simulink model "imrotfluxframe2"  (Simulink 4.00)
settings: Solver=ode45  StartTime=0.0  StopTime=1  MaxStep=2e-4  RelTol=1e-3  AbsTol=1e-3
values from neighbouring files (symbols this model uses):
  an = atan2(phiqr,phidr)    [imdefrotflux.m]
  Bm = 0.10    (= 0.1)    [IMabc2.m]    (also in imabcparam.m = 0.01; IMabcrun0.m = 0.01; IMabcrun1.m = 0.001; IMcur0.m = 1e-06)
  fr0 = [phidr phiqr]    [imdef0vec.m]    (also in imdef1vec.m; imdefrotflux.m = sqrt(phidr^2+phiqr^2); imdefSIvec1.m)
  fs0 = fs    [calc0.m]    (also in imdef0vec.m = [phids phiqs]; imdef1vec.m = [phids phiqs]; imdefrotflux.m = [fs0d fs0q]; imdefSIvec1.m = [phids phiqs])
  H = 0.60    (= 0.6)    [IMabc2.m]    (also in IMcur0.m = 0.3; imdef0vec.m = 0.3; imdef1vec.m = 0.3; imdef2vec.m = 0.3)
  Lm = eval(get(hLm,'String'))    [im3d.m]    (also in IMabc2.m = 4.5; imabcparam.m = 0.0847; IMabcrun0.m = 0.0847; IMabcrun1.m = 0.0847)
  Lrl = eval(get(hLr,'String'))    [im3d.m]    (also in IMabc2.m = 0.1; imabcparam.m = 0.0025; IMabcrun0.m = 0.0025; IMabcrun1.m = 0.0025)
  Lsl = eval(get(hLs,'String'))    [im3d.m]    (also in IMabc2.m = 0.1; imabcparam.m = 0.0025; IMabcrun0.m = 0.0025; IMabcrun1.m = 0.0025)
  n0 = 0.98    [imdef0vec.m]    (also in imdef1vec.m = 0.978; imdef2vec.m; imdefrotflux.m; imdefSIvec1.m = 0.95)
  Rr = input('Rotor resistance)[default = 2] =')    [Actac.m]    (also in im1phase.m = 0.3; im3d.m = eval(get(hRr,'String')); IMabc2.m = 0.02; imabcparam.m = 0.408)
  Rs = eval(get(hRs,'String'))    [im3d.m]    (also in IMabc2.m = 0.01; imabcparam.m = 0.531; IMabcrun0.m = 0.531; IMabcrun1.m = 0.531)
  Tl0 = Is*conj(Is)*Req    [imdef0vec.m]    (also in imdef1vec.m; imdef2vec.m = Lm*(I(2)*I(3)-I(1)*I(4)); imdefrotflux.m; imdefSIvec1.m = Te0/To)
  vs = 1.0    (= 1)    [imdef0vec.m]    (also in imdef1vec.m; imdef2vec.m; imdefrotflux.m; imdefSIvec1.m)
  wo = 2*pi*freq0    [calc0.m]    (also in IMabc2.m = 376.991118431; imabcparam.m = 376.991118431; IMabcrun0.m = 376.991118431; IMabcrun1.m = 376.991118431)
  ws = 1.0    (= 1)    [IMabc2.m]    (also in IMcur0.m; imdef0vec.m; imdef1vec.m; imdef2vec.m)

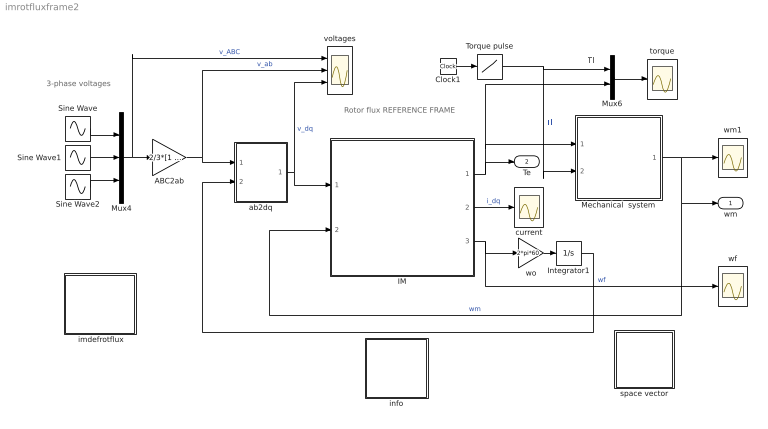
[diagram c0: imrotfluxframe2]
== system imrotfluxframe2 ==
  note: Rotor flux REFERENCE FRAME
  note: Tl
  note: 3-phase voltages
  " imdefrotflux" : Subsystem
  ABC2ab : Gain  Gain=2/3*[1 -0.5 -0.5;0 sqrt(3)/2 -sqrt(3)/2]  Multiplication=Matrix(K*u)  SaturateOnIntegerOverflow=on
  Clock1 : Clock
  IM : Subsystem
  Integrator1 : Integrator  ExternalReset=none  InitialConditionSource=internal  InitialCondition=0  LimitOutput=off  UpperSaturationLimit=inf  LowerSaturationLimit=-inf  ShowSaturationPort=off  ShowStatePort=off  AbsoluteTolerance=auto
  Mechanical  system : Subsystem
  Mux4 : Mux  Inputs=3
  Mux6 : Mux  Inputs=2
  Sine Wave : Sin  Amplitude=vs  Frequency=2*pi*ws*60  Phase=pi/2-an  SampleTime=0
  Sine Wave1 : Sin  Amplitude=vs  Frequency=2*pi*ws*60  Phase=pi/2-an-2*pi/3  SampleTime=0
  Sine Wave2 : Sin  Amplitude=vs  Frequency=2*pi*ws*60  Phase=pi/2-an+2*pi/3  SampleTime=0
  Torque pulse : Lookup  InputValues=[0 0.1 0.1 0.5 0.5 2]  OutputValues="[Tl0 Tl0  0 0 0.5 0.5]"
  ab2dq : Subsystem
  current : Scope
  info : Subsystem
  space vector : Subsystem
  torque : Scope
  voltages : Scope  NumInputPorts=3
  wf : Scope
  wm1 : Scope
  wo : Gain  Gain=2*pi*60  Multiplication=Element-wise(K.*u)  SaturateOnIntegerOverflow=on
  wm : Outport  Port=1
  Te : Outport  Port=2
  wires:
  Mux6/1 -> torque/1
  Torque pulse/1 -> Mux6/1, Mechanical  system/2(Tl)  "Tl"
  Mechanical  system/1(wm) -> wm1/1, IM/2(wm), wm/1  "wm"
  ab2dq/1(dq) -> IM/1(vs), voltages/3  "v_dq"
  Mux4/1 -> ABC2ab/1, voltages/1  "v_ABC"
  ABC2ab/1 -> ab2dq/1(ab), voltages/2  "v_ab"
  IM/2(is) -> current/1  "i_dq"
  IM/1(Te) -> Te/1, Mux6/2, Mechanical  system/1(Te)
  Sine Wave/1 -> Mux4/1
  Sine Wave1/1 -> Mux4/2
  Sine Wave2/1 -> Mux4/3
  Clock1/1 -> Torque pulse/1
  wo/1 -> Integrator1/1
  IM/3(wf) -> wo/1, wf/1  "wf"
  Integrator1/1 -> ab2dq/2(thetak)

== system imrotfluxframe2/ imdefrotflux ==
  note: Double click the block to enter the machine parameters and initial conditions and then run the simulation
  note: This demo simulates the running of an induction motor in steady-state when a sudden input change is effected: a)torque step changes at constant voltage excitation b) voltage input sag at constant frequency and load torque c)simultaneous step changes in voltage magnitude and frequency

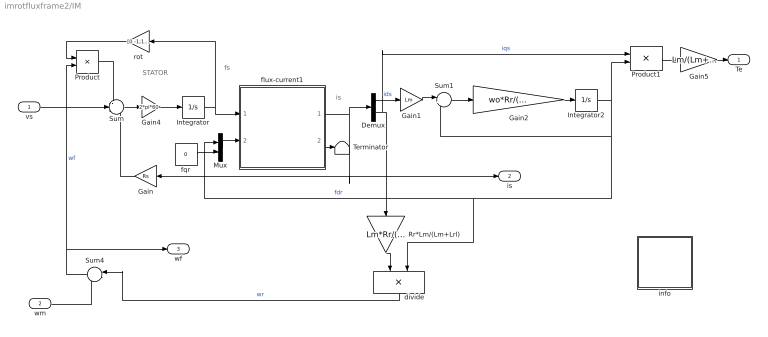
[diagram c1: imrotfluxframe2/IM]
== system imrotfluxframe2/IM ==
  note: STATOR
  note: fs
  note: is
  vs : Inport  Port=1
  wm : Inport  Port=2
  Demux : Demux  Outputs=2  BusSelectionMode=off
  Gain : Gain  Orientation=left  Gain=Rs  Multiplication=Element-wise(K.*u)  SaturateOnIntegerOverflow=on
  Gain1 : Gain  Gain=Lm  Multiplication=Element-wise(K.*u)  SaturateOnIntegerOverflow=on
  Gain2 : Gain  Gain=wo*Rr/(Lm+Lrl)  Multiplication=Element-wise(K.*u)  SaturateOnIntegerOverflow=on
  Gain4 : Gain  Gain=2*pi*60  Multiplication=Element-wise(K.*u)  SaturateOnIntegerOverflow=on
  Gain5 : Gain  Gain=Lm/(Lm+Lrl)  Multiplication=Element-wise(K.*u)  SaturateOnIntegerOverflow=on
  Integrator : Integrator  ExternalReset=none  InitialConditionSource=internal  InitialCondition=fs0  LimitOutput=off  UpperSaturationLimit=inf  LowerSaturationLimit=-inf  ShowSaturationPort=off  ShowStatePort=off  AbsoluteTolerance=auto
  Integrator2 : Integrator  ExternalReset=none  InitialConditionSource=internal  InitialCondition=fr0  LimitOutput=off  UpperSaturationLimit=inf  LowerSaturationLimit=-inf  ShowSaturationPort=off  ShowStatePort=off  AbsoluteTolerance=auto
  Mux : Mux  Inputs=2
  Product : Product  Inputs=2  Multiplication=Element-wise(.*)  SaturateOnIntegerOverflow=on
  Product1 : Product  Inputs=2  Multiplication=Element-wise(.*)  SaturateOnIntegerOverflow=on
  Rr*Lm/(Lm+Lrl) : Gain  Orientation=down  Gain=Lm*Rr/(Lm+Lrl)  Multiplication=Element-wise(K.*u)  SaturateOnIntegerOverflow=on
  Sum : Sum  Inputs=-+-  SaturateOnIntegerOverflow=on
  Sum1 : Sum  Inputs=|+-  SaturateOnIntegerOverflow=on
  Sum4 : Sum  Orientation=left  Inputs=|++  SaturateOnIntegerOverflow=on
  Terminator : Terminator
  divide : Product  Orientation=down  Inputs=*/  Multiplication=Element-wise(.*)  SaturateOnIntegerOverflow=on
  flux-current1 : Subsystem
  fqr : Constant  Value=0
  info : Subsystem
  rot : Gain  Orientation=left  Gain=[0 -1;1 0]  Multiplication=Matrix(K*u)  SaturateOnIntegerOverflow=on
  Te : Outport  Port=1
  is : Outport  Port=2
  wf : Outport  Port=3
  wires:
  Gain/1 -> Sum/3
  Integrator/1 -> flux-current1/1(fs), rot/1
  Product/1 -> Sum/1
  rot/1 -> Product/1
  Sum/1 -> Gain4/1
  Gain4/1 -> Integrator/1
  flux-current1/1(is) -> Gain/1, is/1, Demux/1
  vs/1 -> Sum/2
  wm/1 -> Sum4/2
  Rr*Lm/(Lm+Lrl)/1 -> divide/1
  Demux/1 -> Gain1/1  "ids"
  Sum4/1 -> wf/1, Product/2  "wf"
  divide/1 -> Sum4/1  "wr"
  Mux/1 -> flux-current1/2(fr)
  fqr/1 -> Mux/2
  Demux/2 -> Rr*Lm/(Lm+Lrl)/1, Product1/1  "iqs"
  Gain1/1 -> Sum1/1
  Sum1/1 -> Gain2/1
  Gain2/1 -> Integrator2/1
  Integrator2/1 -> Product1/2, divide/2, Mux/1, Sum1/2  "fdr"
  Product1/1 -> Gain5/1
  Gain5/1 -> Te/1
  flux-current1/2(ir) -> Terminator/1

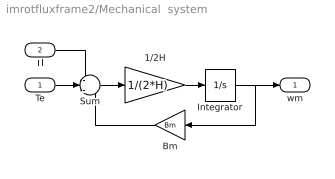
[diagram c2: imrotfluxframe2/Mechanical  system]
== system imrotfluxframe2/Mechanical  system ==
  Te : Inport  Port=1
  Tl : Inport  Port=2
  1/2H : Gain  Gain=1/(2*H)  Multiplication=Element-wise(K.*u)  SaturateOnIntegerOverflow=on
  Bm : Gain  Orientation=left  Gain=Bm  Multiplication=Element-wise(K.*u)  SaturateOnIntegerOverflow=on
  Integrator : Integrator  ExternalReset=none  InitialConditionSource=internal  InitialCondition=n0  LimitOutput=off  UpperSaturationLimit=inf  LowerSaturationLimit=-inf  ShowSaturationPort=off  ShowStatePort=off  AbsoluteTolerance=auto
  Sum : Sum  Inputs=-+-  SaturateOnIntegerOverflow=on
  wm : Outport  Port=1
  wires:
  1/2H/1 -> Integrator/1
  Sum/1 -> 1/2H/1
  Bm/1 -> Sum/3
  Integrator/1 -> Bm/1, wm/1
  Te/1 -> Sum/2
  Tl/1 -> Sum/1

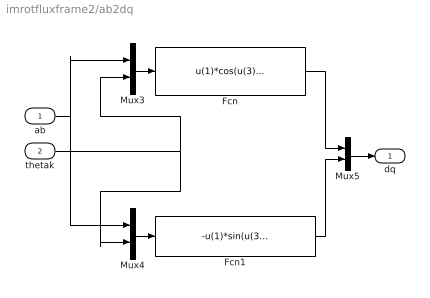
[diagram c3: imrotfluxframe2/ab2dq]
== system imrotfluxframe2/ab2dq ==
  ab : Inport  Port=1
  thetak : Inport  Port=2
  Fcn : Fcn  Expr=u(1)*cos(u(3))+u(2)*sin(u(3))
  Fcn1 : Fcn  Expr=-u(1)*sin(u(3))+u(2)*cos(u(3))
  Mux3 : Mux  Inputs=2
  Mux4 : Mux  Inputs=2
  Mux5 : Mux  Inputs=2
  dq : Outport  Port=1
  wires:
  Mux3/1 -> Fcn/1
  Mux4/1 -> Fcn1/1
  ab/1 -> Mux3/1, Mux4/1
  thetak/1 -> Mux3/2, Mux4/2
  Fcn1/1 -> Mux5/2
  Fcn/1 -> Mux5/1
  Mux5/1 -> dq/1

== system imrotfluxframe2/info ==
  note: Running of an Induction Motor Modeled in the Rotor Flux Frame under Three-Phase Sinusoidal Excitation

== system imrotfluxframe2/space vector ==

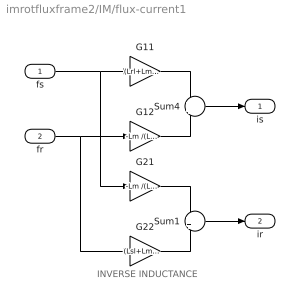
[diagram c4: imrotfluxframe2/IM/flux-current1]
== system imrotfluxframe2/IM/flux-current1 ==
  note: INVERSE INDUCTANCE
  fs : Inport  Port=1
  fr : Inport  Port=2
  G11 : Gain  Gain=(Lrl+Lm) /(Lsl*Lrl+Lsl*Lm+Lrl*Lm)  Multiplication=Element-wise(K.*u)  SaturateOnIntegerOverflow=on
  G12 : Gain  Gain=-Lm /(Lsl*Lrl+Lsl*Lm+Lrl*Lm)  Multiplication=Element-wise(K.*u)  SaturateOnIntegerOverflow=on
  G21 : Gain  Gain=-Lm /(Lsl*Lrl+Lsl*Lm+Lrl*Lm)  Multiplication=Element-wise(K.*u)  SaturateOnIntegerOverflow=on
  G22 : Gain  Gain=(Lsl+Lm )/(Lsl*Lrl+Lsl*Lm+Lrl*Lm)  Multiplication=Element-wise(K.*u)  SaturateOnIntegerOverflow=on
  Sum1 : Sum  Inputs=++  SaturateOnIntegerOverflow=on
  Sum4 : Sum  Inputs=++  SaturateOnIntegerOverflow=on
  is : Outport  Port=1
  ir : Outport  Port=2
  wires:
  fs/1 -> G11/1, G21/1
  G11/1 -> Sum4/1
  fr/1 -> G12/1, G22/1
  G12/1 -> Sum4/2
  Sum4/1 -> is/1
  G21/1 -> Sum1/1
  G22/1 -> Sum1/2
  Sum1/1 -> ir/1

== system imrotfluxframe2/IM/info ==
  note: Mathematical model of the induction machine described in the rotor flux reference frame. (Per unit formulation)
  note: Electrical system equations: vs = Rs.is + 1/wo.(dfs/dt) + j.wk.fs where the variables is, vs, and fs are 2-dimensional space vectors and j represents a 90o space rotator namely j = [0 -1;1 0] wf = wm + wr; wr = Rr. Lm/(Lm+Lrl). (iqs / fdr) 1/wo.(Lm+Lrl)/Rr.(dfdr/dt) +fdr = Lm.ids fqr = 0 The flux linkage current relations : fds = (Lm + Lsl).ids + Lm.idr fdr = Lm.ids + (Lm + Lrl).idr (D_axis) fqs = (Lm + Lsl).iqs + Lm.iqr fqr = Lm.iqs + (Lm+Lrl).iqr (Q_axis) Mechanical system equations: Te = 2H.dwm/dt + Bm.wm + Tl where Te = (iqs.fdr). Lm/(Lm + Lrl)
